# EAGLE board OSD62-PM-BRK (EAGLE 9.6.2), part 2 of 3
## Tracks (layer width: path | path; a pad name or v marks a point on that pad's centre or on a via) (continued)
GPMC0_ADVN_ALE  (via drill 0.1 pad 0.25) (continued)
  Top 0.076: U1.H25 v45.5,14
  Bottom 0.076: v45.5,14 45.75,14.25 46.18,14.25 46.86,14.94 50.14,14.94 52.12,16.92 52.12,21.11 53.49,22.48 56.39,22.48 57.45,23.55 60.73,23.55 61.34,24.16 69.65,24.16 70.87,25.38 75.29,25.38 76.58,26.67 JP4.31
GPMC0_BE0N_CLE  (via drill 0.1 pad 0.25)
  Top 0.076: U1.J26 v46,13.5
  Bottom 0.076: v46,13.5 47.69,13.5 48.23,12.95 50.44,12.95 50.6,12.8 50.6,12.04 48.39,9.83 48.39,7.24 48.92,6.71 55.02,6.71 56.16,5.56 83.13,5.56 83.97,4.72 83.97,3.2 84.51,2.67 93.85,2.67 JP2.38
GPMC0_BE1N  (via drill 0.1 pad 0.25)
  Top 0.076: U1.K25 v45.5,12.5
  Bottom 0.076: v45.5,12.5 45.75,12.25 47.2,12.25 48.08,11.36 48.08,7.09 48.77,6.4 54.86,6.4 56.01,5.26 82.98,5.26 83.67,4.57 83.67,3.05 84.35,2.36 89.08,2.36 JP2.36
GPMC0_CLK  (via drill 0.1 pad 0.25)
  Top 0.076: U1.K26 v46,12.5
  Bottom 0.076: v46,12.5 47.17,12.5 48.23,11.44 48.23,7.16 48.84,6.55 54.94,6.55 56.08,5.41 83.06,5.41 83.82,4.65 83.82,3.12 84.43,2.52 91.47,2.52 JP2.37
GPMC0_CSN0  (via drill 0.1 pad 0.25)
  Top 0.076: U1.F26 v46,15
  Bottom 0.076: v46,15 46.24,15 46.63,15.39 49.91,15.39 51.66,17.14 51.66,21.34 53.26,22.94 56.16,22.94 57.23,24 60.5,24 61.11,24.61 69.42,24.61 71.48,26.67 JP4.29
GPMC0_CSN1  (via drill 0.1 pad 0.25)
  Top 0.076: U1.F25 v45.5,15
  Bottom 0.076: v45.5,15 45.75,15.25 46.26,15.25 46.56,15.54 49.84,15.54 51.51,17.22 51.51,21.41 53.19,23.09 56.08,23.09 57.15,24.16 60.43,24.16 61.04,24.77 69.34,24.77 71.17,26.59 71.17,28.04 72.34,29.21 JP5.29
GPMC0_CSN2  (via drill 0.1 pad 0.25)
  Top 0.076: U1.E26 v46,15.5
  Bottom 0.076: v46,15.5 46.28,15.5 46.48,15.7 49.76,15.7 51.36,17.3 51.36,21.49 53.11,23.24 56.01,23.24 57.07,24.31 60.35,24.31 60.96,24.92 68.12,24.92 69.85,26.64 JP4.28
GPMC0_CSN3  (via drill 0.1 pad 0.25)
  Top 0.076: U1.E25 v45.5,15.5
  Bottom 0.076: v45.5,15.5 45.76,15.76 46.25,15.76 46.34,15.85 49.68,15.85 51.21,17.37 51.21,21.57 53.03,23.39 55.93,23.39 57,24.46 60.27,24.46 60.88,25.07 68.05,25.07 68.66,25.68 68.66,28.04 69.83,29.21 JP5.28
GPMC0_DIR  (via drill 0.1 pad 0.25)
  Top 0.076: U1.G25 v45.5,14.5
  Bottom 0.076: v45.5,14.5 45.75,14.75 46.22,14.75 46.71,15.24 49.99,15.24 51.82,17.07 51.82,21.26 53.34,22.78 56.24,22.78 57.3,23.85 60.58,23.85 61.19,24.46 69.52,24.46 70.74,25.68 72.87,25.68 73.86,26.67 JP4.30
GPMC0_OEN_REN  (via drill 0.1 pad 0.25)
  Top 0.076: U1.H26 v46,14
  Bottom 0.076: v46,14 46.16,14 46.94,14.78 50.22,14.78 52.27,16.84 52.27,21.03 53.57,22.33 56.46,22.33 57.53,23.39 60.81,23.39 61.42,24 69.72,24 70.94,25.22 77.95,25.22 79.4,26.67 JP4.32
GPMC0_WAIT0  (via drill 0.1 pad 0.25)
  Top 0.076: U1.L25 v45.5,12
  Bottom 0.076: v45.5,12 45.75,11.75 47.24,11.75 47.78,11.21 47.78,6.93 48.62,6.1 54.71,6.1 55.85,4.95 80.92,4.95 81.46,4.42 81.46,3.12 81.84,2.74 83.52,2.74 84.99,1.27 JP2.34
GPMC0_WAIT1  (via drill 0.1 pad 0.25)
  Top 0.076: U1.L26 v46,12
  Bottom 0.076: v46,12 47.22,12 47.93,11.29 47.93,7.01 48.69,6.25 54.79,6.25 55.93,5.11 82.91,5.11 83.52,4.5 83.52,2.97 84.28,2.21 86.69,2.21 JP2.35
GPMC0_WEN  (via drill 0.1 pad 0.25)
  Top 0.076: U1.J25 v45.5,13.5
  Bottom 0.076: v45.5,13.5 45.75,13.75 47.67,13.75 48.31,13.11 50.52,13.11 50.75,12.88 50.75,11.96 48.54,9.75 48.54,7.32 49,6.86 55.09,6.86 56.24,5.71 83.21,5.71 84.12,4.8 84.12,3.28 84.58,2.82 96.24,2.82 JP2.39
GPMC0_WPN  (via drill 0.1 pad 0.25)
  Top 0.076: U1.G26 v46,14.5
  Bottom 0.076: v46,14.5 46.2,14.5 46.79,15.09 50.06,15.09 51.97,16.99 51.97,21.18 53.42,22.63 56.31,22.63 57.38,23.7 60.66,23.7 61.27,24.31 69.58,24.31 70.8,25.53 75.21,25.53 76.12,26.44 76.12,28.73 76.61,29.21 JP5.31
I2C0_SCL  (via drill 0.1 pad 0.25, 0.25 pad 0.46)
  Top 0.076: U1.A12 38.75,17.95 39.7,18.9 v40.08,18.9 40.23,18.75 40.84,18.75 42.14,20.04 42.14,20.65 44.27,22.78 51.51,22.78 54.86,19.43 v54.86,19.2 | v74.45,19.96 73.96,20.45 U4.1 | U8.5 77.47,19.75 76.92,19.2 76.05,19.2 75.82,19.43 v75.82,19.96 | v15.47,4.72 14.71,4.72 14.25,5.18 14.25,7.85 14.1,8 v13.64,8
  Top 0.127: U6.10 14.75,12.17 14.35,12.57 v14.35,13.21 14.1,13.46 13.84,13.46 13.72,13.34 13.72,13.03 R52.1 | U7.5 2.46,7.95 2.41,8 2.41,9.4 v2.67,9.65
  Bottom 0.076: v40.08,18.9 39.85,18.9 38.1,20.65 22.55,20.65 20.19,18.29 20.19,16.38 19.74,15.93 15.24,15.93 14.78,15.47 14.78,14.02 14.35,13.59 v14.35,13.21 | v54.86,19.2 54.86,19.81 55.17,20.12 74.3,20.12 v74.45,19.96 74.6,20.12 75.67,20.12 v75.82,19.96 75.97,20.12 97.46,20.12 99.14,21.79 99.14,23.93 99.34,24.13 J7.2 | v14.35,13.21 14.35,12.83 13.34,11.81 13.34,8.31 v13.64,8 | v15.47,4.72 15.67,4.93 20.02,4.93 20.27,5.18 20.27,5.41 19.96,5.72 J8.2 | v14.35,13.21 12.9,13.21 11.12,11.43 8,11.43 7.77,11.66 4.42,11.66 3.96,11.2 3.96,9.6 3.58,9.22 3.1,9.22 v2.67,9.65
I2C0_SDA  (via drill 0.1 pad 0.25, 0.25 pad 0.46)
  Top 0.076: U1.B12 38.5,17 38.5,17.93 39.78,19.2 40.31,19.2 v40.46,19.05 40.62,18.9 40.77,18.9 41.99,20.12 41.99,20.73 44.2,22.94 51.59,22.94 55.17,19.36 55.17,19.13 v54.86,18.82 | U4.3 71.92,20.42 v71.4,20.42 | v75.82,20.42 76.3,20.42 U8.6 | v15.47,4.34 14.86,4.34 14.1,5.11 14.1,7.54 v13.95,7.7
  Top 0.127: U6.9 15.11,12.69 15.11,13.21 v14.77,13.55 v14.35,13.97 R53.1 | U7.6 3.3,8.94 v3.3,9.65
  Bottom 0.076: v40.46,19.05 40.31,19.2 39.78,19.2 38.18,20.8 22.48,20.8 20.04,18.36 20.04,16.46 19.66,16.08 15.16,16.08 14.63,15.54 14.63,14.25 v14.35,13.97 13.44,13.97 11.05,11.58 8.08,11.58 7.85,11.81 4.34,11.81 3.81,11.28 3.81,10.16 v3.3,9.65 | v54.86,18.82 54.56,19.13 54.56,19.96 54.86,20.27 71.25,20.27 v71.4,20.42 71.55,20.27 75.67,20.27 v75.82,20.42 75.97,20.27 97.38,20.27 98.98,21.87 98.98,23.93 98.78,24.13 J7.1 | v14.77,13.55 14.77,13.02 13.49,11.73 13.49,8.53 13.95,8.08 v13.95,7.7 | v15.47,4.34 15.9,4.78 20.1,4.78 20.43,5.1 20.43,6.46 J8.3
I2C1_SCL
  Top 0.076: JP3.36 91.31,4.95 93.34,4.95 93.65,5.26 96.01,5.26 96.55,5.79 96.55,6.93 93.42,10.06 87.94,10.06 87.33,10.67 87.33,18.44 86.49,19.28 81.08,19.28 80.24,18.44 80.24,16.69 79.7,16.15 56.39,16.15 54.41,18.14 54.41,19.43 51.36,22.48 44.42,22.48 42.44,20.5 42.44,19.89 41,18.44 39.7,18.44 39.25,17.99 U1.A13
  Bottom 0.127: JP3.36 R69.1
I2C1_SDA
  Top 0.076: JP3.35 88.77,2.67 90.91,2.67 91.44,3.2 91.44,4.12 92.13,4.8 93.42,4.8 93.73,5.11 96.09,5.11 96.7,5.71 96.7,7.01 93.5,10.21 88.01,10.21 87.48,10.74 87.48,18.52 86.56,19.43 81,19.43 80.09,18.52 80.09,16.76 79.63,16.31 56.46,16.31 54.56,18.21 54.56,19.51 51.44,22.63 44.35,22.63 42.29,20.57 42.29,19.96 40.92,18.59 39.62,18.59 39,17.97 39,17 U1.B13
  Bottom 0.127: JP3.35 R70.1
LDO1-1P8-3P3  (via drill 0.1 pad 0.25, 0.25 pad 0.46)
  Top 0.152: U1.G21 v43.5,14.5 | U1.G22 v44,14.5
  Top 0.254: U6.7 16.28,13.57 v15.62,14.22 15.11,14.73 C42.1 | R43.2 95.17,5.84 94.31,5.84 R44.2 94.16,5.84 93.29,5.84 R45.2 93.22,5.46 92.96,5.21 91.44,5.21 91.19,5.46 R46.2 91.11,5.84 90.25,5.84 R47.2 90.17,5.46 89.66,4.95 87.38,4.95 v86.74,5.59 | v66.06,8.08 65.35,7.37 59.56,7.37 59.05,7.87 53.72,7.87 50.04,11.56 50.04,11.86 C23.1 49.66,11.94 v49.4,12.19
  Route15 0.076: v44,14.5 43.88,14.5 43.75,14.62 43.75,15.12 43.62,15.25 42.38,15.25 42.12,15 | 42.12,15 42.38,14.75 43.25,14.75 v43.5,14.5 U1.G21 42.38,14.25 42.12,14.5 42.12,15
  Route15 0.254: v33.1,17.78 33.1,17.42 33.68,16.84 38.81,16.84 39.37,17.4 39.63,17.4 39.88,17.15 39.88,15.25 40.12,15 42.12,15
  Bottom 0.254: v43.5,14.5 v44,14.5 44.62,13.88 44.62,13.25 44.88,13 47.2,13 48.01,12.19 v49.4,12.19 | v15.62,14.22 16.71,15.32 19.96,15.32 22.85,18.2 32.23,18.2 32.65,17.78 v33.1,17.78 | v86.74,5.59 83.82,5.59 80.77,8.64 66.62,8.64 v66.06,8.08
  pour Route15: 43.38,14.38 43.38,14.62 44.12,14.62 44.12,14.38
LDO2-0P85  (via drill 0.1 pad 0.25, 0.25 pad 0.46)
  Top 0.076: C18.1 15.39,8.76 15.57,8.94 16.67,8.94 16.78,8.83 U6.19
  Top 0.152: U1.K17 v41.5,12.5 | U1.L17 v41.5,12 | U1.L18 v42,12 | U1.K18 v42,12.5 | U1.H17 v41.5,14 | U1.J17 v41.5,13.5 | U1.J18 v42,13.5 | U1.H18 v42,14 | v20.73,5.77 20.88,5.92 21,5.92 C17.1 | C19.1 40.16,7.39 v40.01,7.54
  Top 0.254: C43.1 15.75,7.49 15.88,7.62 v16.26,7.62 16.78,8.14 U6.19
  Route15 0.152: v20.73,5.77 20.73,6.38
  Route15 0.381: v16.26,7.62 17.5,6.38 19.94,6.38 20.73,6.38 34.19,6.38 37.34,9.53 38.86,9.53 41.34,12 v41.5,12
  Bottom 0.152: v41.5,12 41.16,11.66 40.39,11.66 40.16,11.89 39.85,11.89 39.62,11.66 39.62,11.35 39.78,11.2 39.78,10.75 39.17,10.13 39.17,7.71 39.49,7.39 39.85,7.39 v40.01,7.54
  pour Route15: 41.38,14.12 41.38,12.25 40.62,11.5 41.62,11.5 42.12,12 42.12,14.12
LDO3-1P8  (via drill 0.1 pad 0.25, 0.25 pad 0.46)
  Top 0.076: U1.D15 v40.5,16
  Top 0.127: R24.2 14.73,6.35 14.86,6.48 17.65,6.48 | 17.78,6.6 17.65,6.48 | 17.78,6.6 C44.1 | Y1.4 29.11,17.88 28.7,18.29 28.7,18.31 C46.1 | 17.78,6.6 17.91,6.48 | C5.1 21.29,6.48 17.91,6.48 | 17.65,6.48 17.91,6.48
  Top 0.152: U1.P11 v38,10.5 | U1.N12 v38.5,11 | U1.N13 v39,11 | U1.P12 v38.5,10.5 | U1.P13 v39,10.5 | U1.N14 v39.5,11 | U1.F13 v39,15 | U1.F14 v39.5,15 | v24.08,19.81 24.69,19.2 24.69,16.92 v24.92,16.69 | 28.7,18.31 28.63,18.39 28.6,18.36 27.61,18.36 27.2,18.77 v27.2,19.81 27.2,20.8 | 27.2,20.8 27.64,20.8 R50.1 27.74,20.8 28.83,20.8 Y2.4 | 27.2,20.8 26.72,20.8 C54.1 | C3.1 39.78,18.14 v39.62,17.98 | C4.1 29.72,7.49 | 29.72,7.49 v29.72,7.47 | C1.1 30.48,7.92 30.05,7.49 29.72,7.49 | C2.1 41.07,7.39 v41.22,7.54
  Top 0.254: C44.1 v17.78,7.67 U6.21
  Route15 0.381: v38.5,10.5 38.03,10.03 37.16,10.03 34.01,6.88 30.91,6.88 30.33,7.47 v29.72,7.47 29.11,7.47 28.52,6.88 18.26,6.88 17.78,7.37 v17.78,7.67
  Bottom 0.152: v39,15 v39.5,15 39.75,15 40.5,15.75 v40.5,16 40,16.5 40,17.45 39.62,17.83 | v24.08,19.81 v27.2,19.81 37.64,19.81 39.47,17.98 | v24.92,16.69 23.39,16.69 22.4,15.7 22.4,13.41 21.26,12.27 19.58,12.27 18.75,11.43 16.38,11.43 16,11.05 16,8.43 16.64,7.8 16.64,7.52 16.99,7.16 17.27,7.16 v17.78,7.67 | v39,10.5 38.92,10.42 38.92,7.63 39.4,7.16 40.84,7.16 v41.22,7.54 | 39.47,17.98 v39.62,17.98 39.62,17.83 | 39.47,17.98 39.62,17.83
  pour Route15: 38.5,11.12 37.28,9.91 38.66,9.91 39.88,11.12
LDO4-2P5  (via drill 0.1 pad 0.25, 0.25 pad 0.46)
  Top 0.152: U1.N10 v37.5,11 | C20.1 v30.35,11.56
  Top 0.254: U6.23 18.78,8.28 v19.43,7.62 19.68,7.62 19.81,7.49 C45.1
  Route15 0.254: v37.5,11 37.5,10.98 33.83,7.32 31.09,7.32 30.48,7.92 28.96,7.92 28.35,7.32 19.74,7.32 v19.43,7.62
  Bottom 0.076: v37.5,11 37.25,11.25 33.8,11.25 33.3,10.74 32.54,10.74 31.73,11.56 v30.35,11.56
LED1
  Top 0.127: R57.1 3.25,21.08 2.27,21.08 D1.1
LED2
  Top 0.076: R58.1 82.68,16.76 82.45,16.54 82.22,16.54 81.61,15.93 81.61,11.94 81.86,11.68 D2.1
LED3
  Top 0.076: R59.1 81.66,16.2 81.46,16 81.46,10.11 81.79,9.78 D3.1
LED4
  Top 0.076: R60.1 83.69,16.64 83.44,16.38 82.3,16.38 81.76,15.85 81.76,13.72 81.89,13.59 D4.1
LED5
  Top 0.076: D5.1 82.44,16.07 82.6,16.23 84.35,16.23 84.71,16.59 R61.1
LX_B1
  pour Top (no thermals): 18.16,13.08 18.16,13.97 19.05,14.86 19.05,16.13 20.07,16.13 20.07,14.22 19.43,14.22 18.92,13.72 18.92,13.08
LX_B2
  pour Top (no thermals): 19.68,11 21.84,11 21.84,12.06 21.03,12.06 21.03,11.33 19.68,11.33
LX_B3
  pour Top (no thermals): 19.68,10.34 21.84,10.34 21.84,9.27 21.01,9.27 21.01,10.06 19.68,10.06
MCAN0_RX
  Top 0.076: U1.A11 38.25,17.91 39.7,19.36 40.98,19.36 41.83,20.21 41.83,20.8 44.12,23.09 51.66,23.09 58.29,16.46 79.55,16.46 79.93,16.84 79.93,18.59 80.92,19.58 86.64,19.58 87.63,18.59 87.63,10.82 88.09,10.36 93.57,10.36 96.85,7.09 96.85,5.64 96.16,4.95 93.8,4.95 92.71,3.86 JP3.37
MCAN0_TX
  Top 0.076: U1.B11 38,17 38,17.88 39.62,19.51 40.92,19.51 41.68,20.27 41.68,20.88 44.04,23.24 51.74,23.24 58.37,16.61 79.48,16.61 79.78,16.92 79.78,18.67 80.85,19.74 86.72,19.74 87.78,18.67 87.78,10.9 88.16,10.52 93.65,10.52 97,7.16 97,5.56 JP3.38
MCASP0_ACLKR  (via drill 0.1 pad 0.25)
  Top 0.076: U1.B19 42.5,17 42.5,17.66 43.81,18.97 43.81,19.81 44.81,20.8 50.37,20.8 55.93,15.24 80.09,15.24 81.15,14.17 81.15,9.6 81.69,9.07 93.95,9.07 95.78,7.24 v95.78,5.79
  Bottom 0.076: v95.78,5.79 97.77,3.81 JP3.39
MCASP0_ACLKX
  Top 0.076: U1.A18 41.75,17.59 43.36,19.2 43.36,20.04 44.58,21.26 50.6,21.26 56.16,15.7 79.93,15.7 80.7,16.46 80.7,18.21 81.31,18.82 82.58,18.82 82.68,18.72 R58.2
MCASP0_AFSR  (via drill 0.1 pad 0.25)
  Top 0.076: v96.09,6.1 95.94,6.25 95.94,7.32 95.86,7.39 94.03,9.22 81.76,9.22 81.31,9.68 81.31,14.25 80.16,15.39 56.01,15.39 50.44,20.95 44.73,20.95 43.66,19.89 43.66,19.05 42.25,17.64 U1.A19
  Bottom 0.076: v96.09,6.1 96.09,5.71 96.85,4.95 99.19,4.95 JP3.40
MCASP0_AFSX
  Top 0.076: U1.B18 42,17 42,17.62 43.51,19.13 43.51,19.96 44.65,21.11 50.52,21.11 56.08,15.54 80.01,15.54 80.85,16.38 80.85,17.98 81.2,18.34 R59.2
MCASP0_AXR0
  Top 0.076: U1.B17 41.5,17 41.5,17.57 43.2,19.28 43.2,20.12 44.5,21.41 50.67,21.41 56.24,15.85 79.86,15.85 80.54,16.54 80.54,18.29 81.23,18.97 83.52,18.97 83.69,18.8 R60.2
MCASP0_AXR1
  Top 0.076: U1.A17 41.25,17.55 43.05,19.36 43.05,20.19 44.42,21.57 50.75,21.57 56.31,16 79.78,16 80.39,16.61 80.39,18.36 81.15,19.13 84.43,19.13 84.71,18.85 R61.2
MCASP0_AXR2  (via drill 0.1 pad 0.25)
  Top 0.076: U1.B16 41,17 41,17.53 42.9,19.43 42.9,20.27 44.35,21.72 50.83,21.72 53.65,18.9 v53.8,18.9
  Bottom 0.076: v53.8,18.9 53.65,19.05 53.65,19.89 54.48,20.73 69.42,20.73 71.63,22.94 84.35,22.94 86.64,25.22 94.03,25.22 94.41,25.6 96.77,25.6 97.79,26.62 JP4.39
MCASP0_AXR3  (via drill 0.1 pad 0.25)
  Top 0.076: v54.1,18.67 54.1,18.97 51.21,21.87 44.27,21.87 42.75,20.34 42.75,19.51 40.75,17.51 U1.A16 | v95.91,25.3 95.91,24.71 R55.1
  Bottom 0.076: v54.1,18.67 54.1,18.97 53.8,19.28 53.8,19.81 54.56,20.57 69.49,20.57 71.7,22.78 84.43,22.78 86.72,25.07 94.11,25.07 94.49,25.45 95.76,25.45 v95.91,25.3
MCU_ERRORN  (via drill 0.1 pad 0.25)
  Top 0.076: U1.D7 v36,16
  Bottom 0.076: TP2.TP U1.D7 v36,16
MCU_I2C0_SCL  (via drill 0.1 pad 0.25)
  Top 0.076: U1.A7 36.25,17.39 35.74,17.91 35.74,22.86 35.94,23.06 35.94,23.37 36.14,23.57 R65.1 36.45,24 36.32,24.13 v35.94,24.13
  Bottom 0.076: v35.94,24.13 35.74,24.33 35.74,27.76 JP5.14
MCU_I2C0_SDA  (via drill 0.1 pad 0.25)
  Top 0.076: U1.B7 36,17 36,17.42 35.59,17.83 35.59,22.94 35.43,23.09 R66.1 v35.43,24.13
  Bottom 0.076: v35.43,24.13 35.13,24.43 35.13,25.83 JP4.14
MCU_MCAN0_RX
  Top 0.076: U1.E1 32.75,15.25 31.93,16.07 31.93,21.34 31.55,21.72 25.15,21.72 22.1,24.77 19.28,24.77 17.91,26.14 17.91,27.28 17.22,27.96 15.85,27.96 15.7,28.12 13.34,28.12 13.18,28.27 10.9,28.27 9.96,29.21 JP5.4
MCU_MCAN0_TX
  Top 0.076: U1.E2 33.5,15.5 32.75,15.5 32.08,16.17 32.08,21.41 31.62,21.87 25.22,21.87 22.17,24.92 19.36,24.92 18.06,26.21 18.06,27.36 17.3,28.12 15.93,28.12 15.77,28.27 13.41,28.27 12.47,29.21 JP5.5
MCU_MCAN1_RX
  Top 0.076: U1.F1 32.75,14.75 31.62,15.88 31.62,21.18 31.39,21.41 24.99,21.41 21.95,24.46 19.13,24.46 17.6,25.98 17.6,27.13 17.07,27.66 15.7,27.66 15.54,27.81 13.18,27.81 13.03,27.96 5.11,27.96 3.86,29.21 JP5.2
MCU_MCAN1_TX
  Top 0.076: U1.F2 33.5,15 32.75,15 31.77,15.97 31.77,21.26 31.47,21.57 25.07,21.57 22.02,24.61 19.2,24.61 17.75,26.06 17.75,27.2 17.14,27.81 15.77,27.81 15.62,27.96 13.26,27.96 13.11,28.12 7.47,28.12 6.38,29.21 JP5.3
MCU_OSC0_XI
  Top 0.076: U1.G1 32.84,14.25 31.39,15.7 31.39,20.34 30.94,20.8 30.35,20.8 Y2.3
MCU_PORZ  (via drill 0.1 pad 0.25)
  Top 0.076: U1.D6 v35.5,16 | v35.33,18.29 35.43,18.39 35.43,22.39 v35.34,22.48
  Top 0.127: U6.18 16.28,8.15 16.13,8 14.99,8 v14.73,7.75 R24.1
  Bottom 0.076: v35.5,16 35.25,16.25 35.25,17.98 35.33,18.06 v35.33,18.29 35.18,18.44 22.71,18.44 19.89,15.62 15.47,15.62 15.24,15.39 15.24,12.88 14.73,12.37 v14.73,7.75 | 36.42,26.26 JP4.15 36.04,25.88 36.04,25.22 36.42,24.84 36.42,22.78 36.12,22.48 v35.34,22.48
MCU_RESETSTATZ  (via drill 0.1 pad 0.25)
  Top 0.076: U1.C6 v35.5,16.5
  Bottom 0.076: TP3.TP 35.62,15 35.75,15.12 U1.C6 v35.5,16.5
MCU_RESETZ  (via drill 0.1 pad 0.25)
  Top 0.076: U1.C5 v35,16.5 | v33.68,17.83 33.53,17.83 33.4,17.96 R10.1
  Bottom 0.076: v35,16.5 35,17.27 34.44,17.83 v33.68,17.83
MCU_SPI0_CLK
  Top 0.076: U1.A4 34.75,17.52 34.44,17.83 34.44,24.77 34.14,25.07 32.46,25.07 32.31,25.22 28.12,25.22 JP4.11
MCU_SPI0_CS0
  Top 0.076: U1.B6 35.5,17 35.5,17.46 34.9,18.06 34.9,24.99 34.37,25.53 32.69,25.53 32.54,25.68 31.24,25.68 30.63,26.29 30.63,28.09 JP5.13
MCU_SPI0_CS1
  Top 0.076: U1.A6 35.75,17.44 35.05,18.14 35.05,25.07 34.44,25.68 32.77,25.68 31.77,26.67 JP4.13
MCU_SPI0_D0
  Top 0.076: U1.B5 35,17 35,17.5 34.59,17.91 34.59,24.84 34.21,25.22 32.54,25.22 32.38,25.38 28.88,25.38 28.12,26.14 28.12,28.12 JP5.12
MCU_SPI0_D1
  Top 0.076: U1.A5 35.25,17.48 34.75,17.98 34.75,24.92 34.29,25.38 32.61,25.38 32.46,25.53 30.33,25.53 29.21,26.64 JP4.12
MCU_UART0_CTSN
  Top 0.076: U1.B4 34.5,17 34.5,17.55 34.29,17.75 34.29,21.26 32.46,23.09 25.83,23.09 25.38,23.55 25.38,27.91 JP5.11
MCU_UART0_RTSN
  Top 0.076: U1.A3 34.25,17.57 34.14,17.68 34.14,21.18 32.38,22.94 25.76,22.94 24.13,24.56 JP4.10
MCU_UART0_RXD
  Top 0.076: U1.B2 32.84,17.66 32.84,21.79 32,22.63 25.6,22.63 21.59,26.64 JP4.9
MCU_UART0_TXD
  Top 0.076: U1.B3 34,17 34,17.59 33.98,17.6 33.98,21.11 32.31,22.78 25.68,22.78 23.01,25.45 23.01,28.09 JP5.10
MDIO0_MDC
  Top 0.076: JP3.12 30.35,2.67 44.88,2.67 45.75,3.54 U1.V26
MDIO0_MDIO
  Top 0.076: U1.U26 46,9 46,3.56 44.96,2.52 30.45,2.52 JP2.12
MMC0_CLK
  Top 0.076: JP4.5 12.42,27.66 14.86,27.66 15.24,27.28 15.24,26.06 15.77,25.53 17.83,25.53 19.05,24.31 21.87,24.31 26.14,20.04 26.14,18.44 29.87,14.71 31.47,14.71 32.93,13.25 U1.J1
  Bottom 0.127: R67.1 JP4.5
MMC0_CMD
  Top 0.076: U1.K1 33.02,12.75 32.97,12.8 31.55,12.8 25.98,18.36 25.98,19.96 21.79,24.16 18.97,24.16 17.75,25.38 15.24,25.38 13.97,26.64 JP4.6
  Bottom 0.127: R68.1 JP4.6
MMC0_DAT0  (via drill 0.1 pad 0.25)
  Top 0.076: U1.K2 33.5,12.5 32.99,12.5 32.84,12.65 32.69,12.65 v32.38,12.34
  Bottom 0.076: JP3.4 9.98,3.81 11.12,4.95 14.63,4.95 15.47,5.79 15.47,12.19 16.08,12.8 20.34,12.8 21.87,14.33 21.87,15.93 23.24,17.3 27.43,17.3 27.89,16.84 31.93,16.84 32.23,16.54 32.23,12.5 v32.38,12.34
MMC0_DAT1  (via drill 0.1 pad 0.25)
  Top 0.076: v32.77,12.34 32.99,12.34 33.09,12.25 U1.L1
  Bottom 0.076: JP3.3 7.34,4.8 10.74,4.8 11.05,5.11 14.55,5.11 15.32,5.87 15.32,12.27 16,12.95 20.27,12.95 21.72,14.4 21.72,16 23.16,17.45 27.51,17.45 27.96,16.99 32,16.99 32.38,16.61 32.38,12.72 v32.77,12.34
MMC0_DAT2
  Top 0.076: U1.L2 33.5,12 33.03,12 32.99,12.04 32.08,12.04 25.83,18.29 25.83,19.89 21.72,24 18.9,24 17.68,25.22 10.82,25.22 10.13,25.91 10.13,27.36 9.68,27.81 3.5,27.81 2.36,26.67 JP4.1
MMC0_DAT3
  Top 0.076: U1.M1 33.06,11.75 32.92,11.89 32,11.89 25.68,18.21 25.68,19.81 21.64,23.85 18.82,23.85 17.6,25.07 10.74,25.07 9.98,25.83 9.98,27.28 9.6,27.66 4.88,27.66 3.89,26.67 JP4.2
MMC0_DAT4  (via drill 0.1 pad 0.25)
  Top 0.076: U1.M2 33.5,11.5 33.08,11.5 32.84,11.73 32.61,11.73 v32.46,11.58
  Bottom 0.076: JP3.6 15.77,5.61 15.77,12.04 16.23,12.5 20.5,12.5 22.17,14.17 22.17,15.77 23.39,16.99 27.28,16.99 27.74,16.54 31.77,16.54 31.93,16.38 31.93,12.12 v32.46,11.58
MMC0_DAT5  (via drill 0.1 pad 0.25)
  Top 0.076: v32.77,11.35 32.87,11.25 U1.N1
  Bottom 0.076: JP3.5 12.42,4.8 14.71,4.8 15.62,5.71 15.62,12.12 16.15,12.65 20.42,12.65 22.02,14.25 22.02,15.85 23.32,17.14 27.36,17.14 27.81,16.69 31.85,16.69 32.08,16.46 32.08,12.19 32.38,11.89 32.54,11.89 32.77,11.66 v32.77,11.35
MMC0_DAT6
  Top 0.076: U1.N2 33.5,11 32.66,11 25.53,18.14 25.53,19.74 21.57,23.7 18.75,23.7 17.53,24.92 10.67,24.92 8.91,26.67 JP4.4
MMC0_DAT7
  Top 0.076: U1.P1 32.68,10.75 25.38,18.06 25.38,19.66 21.49,23.55 18.67,23.55 17.45,24.77 9.22,24.77 7.32,26.67 JP4.3
MMC1_CLK
  Top 0.076: U1.B21 43.5,17 43.5,17.59 44.42,18.52 44.42,19.51 45.11,20.19 50.06,20.19 55.63,14.63 79.78,14.63 80.54,13.87 80.54,9.3 81.38,8.46 90.75,8.46 91.67,7.54 91.67,6.1 91.85,5.92 R33.2
MMC1_CLK_R  (via drill 0.1 pad 0.25, 0.25 pad 0.46)
  Top 0.076: R33.1 v92.2,6.48
  Top 0.127: 96.42,12.7 95.38,12.7 95.25,12.83 95.25,13.21 95.12,13.34 94.74,13.34 94.61,13.21 94.61,12.83 94.49,12.7 94.11,12.7 93.98,12.83 93.98,13.21 93.85,13.34 93.47,13.34 93.34,13.21 93.34,12.83 93.22,12.7 92.84,12.7 92.71,12.83 92.71,13.21 92.58,13.34 92.2,13.34 92.08,13.21 92.08,12.83 91.95,12.7 v91.69,12.7
  Top 0.152: X1.PIN5 96.42,12.7
  Bottom 0.127: v91.69,12.7 91.69,6.99 v92.2,6.48
MMC1_CMD  (via drill 0.1 pad 0.25, 0.25 pad 0.46)
  Top 0.076: U1.A21 43.25,17.57 44.27,18.59 44.27,19.58 45.03,20.34 50.14,20.34 55.7,14.78 79.86,14.78 80.7,13.95 80.7,9.37 81.46,8.61 92.2,8.61 93.22,7.59 R45.1 v93.22,6.48
  Top 0.127: X1.PIN3 95.38,14.99 95.25,15.11 95.25,15.49 95.12,15.62 94.74,15.62 94.61,15.49 94.61,15.11 94.49,14.99 94.11,14.99 93.98,15.11 93.98,15.49 93.85,15.62 93.47,15.62 93.34,15.49 93.34,15.11 93.22,14.99 v92.2,14.99
  Bottom 0.127: v92.2,14.99 92.71,14.48 92.71,6.99 v93.22,6.48
MMC1_DAT0  (via drill 0.1 pad 0.25, 0.25 pad 0.46)
  Top 0.076: U1.A22 43.75,17.61 44.58,18.44 44.58,19.43 45.19,20.04 49.99,20.04 55.55,14.48 79.7,14.48 80.39,13.79 80.39,9.22 81.31,8.31 90.45,8.31 91.19,7.57 R46.1 v91.19,6.48
  Top 0.127: X1.PIN7 96.46,10.54 95.5,10.54 95.25,10.79 95.25,12.32 95.12,12.45 94.74,12.45 94.61,12.32 94.61,11.94 94.49,11.81 94.11,11.81 93.98,11.94 93.98,12.32 93.85,12.45 93.47,12.45 93.34,12.32 93.34,11.94 93.22,11.81 92.84,11.81 92.71,11.94 92.71,12.32 92.58,12.45 92.2,12.45 92.08,12.32 92.08,11.94 91.95,11.81 91.57,11.81 90.68,12.7 v90.68,13.08
  Bottom 0.127: v90.68,13.08 90.68,6.73 90.93,6.48 v91.19,6.48
MMC1_DAT1  (via drill 0.1 pad 0.25, 0.25 pad 0.46)
  Top 0.076: U1.B22 44,17 44,17.64 44.73,18.36 44.73,19.36 45.26,19.89 49.91,19.89 55.47,14.33 79.63,14.33 80.24,13.72 80.24,9.14 81.23,8.15 89.61,8.15 90.17,7.59 R47.1 90.17,6.6 90.04,6.48 v89.66,6.48
  Top 0.127: X1.PIN8 96.45,9.53 95.5,9.53 94.61,10.41 94.61,11.43 94.49,11.56 94.11,11.56 93.98,11.43 93.98,10.92 93.85,10.79 93.47,10.79 93.34,10.92 93.34,11.43 93.22,11.56 92.84,11.56 92.71,11.43 92.71,10.92 92.58,10.79 92.2,10.79 92.08,10.92 92.08,11.43 91.95,11.56 91.57,11.56 91.44,11.43 91.44,10.92 91.31,10.79 90.93,10.79 90.81,10.92 90.81,11.94 90.68,12.06 90.3,12.06 90.17,11.94 90.17,11.05 90.04,10.92 v89.66,10.92
  Bottom 0.127: v89.66,10.92 v89.66,6.48
MMC1_DAT2  (via drill 0.1 pad 0.25, 0.25 pad 0.46)
  Top 0.076: v95.25,6.48 R43.1 95.25,7.54 93.88,8.91 81.61,8.91 81,9.53 81,14.1 80.01,15.09 55.85,15.09 50.29,20.65 44.88,20.65 43.97,19.74 43.97,18.75 42.75,17.53 U1.A20
  Top 0.127: v94.74,17.27 96.4,17.27 X1.PIN1
  Bottom 0.127: v95.25,6.48 94.74,6.99 v94.74,17.27
MMC1_DAT3  (via drill 0.1 pad 0.25, 0.25 pad 0.46)
  Top 0.076: U1.B20 43,17 43,17.55 44.12,18.67 44.12,19.66 44.96,20.5 50.22,20.5 55.78,14.94 79.93,14.94 80.85,14.02 80.85,9.45 81.53,8.76 93.04,8.76 94.23,7.57 R44.1 v94.23,6.48
  Top 0.127: X1.PIN2 96.25,16.13 95.38,16.13 95.25,16.26 95.25,16.51 95.12,16.64 94.74,16.64 94.61,16.51 94.61,16.26 94.49,16.13 v93.73,16.13
  Bottom 0.127: v93.73,16.13 93.73,6.99 v94.23,6.48
MMC1_SDCD
  Top 0.076: U1.A23 44.25,17.66 44.88,18.29 44.88,19.28 45.34,19.74 49.84,19.74 55.4,14.17 79.4,14.17 80.09,13.49 80.09,9.07 81.15,8 88.85,8 89.25,7.6 U11.4
MMC1_SDWP  (via drill 0.1 pad 0.25)
  Top 0.076: U1.B23 44.5,17 44.5,17.37 v46.1,18.97 | R13.1 13.23,10.92 13.11,11.05 13.11,14.25 13.41,14.55 v14.33,14.55
  Top 0.127: U6.12 14.48,11.18 14.22,11.43 13.84,11.43 13.72,11.3 13.72,11 R13.1
  Bottom 0.076: v14.33,14.55 14.48,14.71 14.48,15.62 15.09,16.23 19.2,16.23 19.43,16.46 19.43,18.21 22.33,21.11 37.57,21.11 38.02,21.57 38.02,24.99 38.48,25.45 42.9,25.45 43.59,24.77 46.48,24.77 46.86,24.38 46.86,20.04 46.1,19.28 v46.1,18.97
MMC2_CLK  (via drill 0.1 pad 0.25)
  Top 0.076: U1.D23 v44.5,16
  Bottom 0.076: v44.5,16 44.75,16.25 44.75,16.79 45.19,17.22 47.62,17.22 48.39,17.98 48.39,25.53 JP4.20
MMC2_CMD  (via drill 0.1 pad 0.25)
  Top 0.076: U1.C23 v44.5,16.5
  Bottom 0.076: v44.5,16.5 44.5,16.84 45.41,17.75 47.32,17.75 48.23,18.67 48.23,28.04 49.4,29.21 JP5.20
MMC2_DAT0  (via drill 0.1 pad 0.25)
  Top 0.076: U1.D22 v44,16
  Bottom 0.076: v44,16 44.25,16.25 44.25,16.82 45.34,17.91 47.24,17.91 48.08,18.75 48.08,28.04 46.99,29.13 JP5.19
MMC2_DAT1  (via drill 0.1 pad 0.25)
  Top 0.076: U1.C22 v44,16.5
  Bottom 0.076: v44,16.5 44,16.8 45.26,18.06 47.17,18.06 47.93,18.82 47.93,25.73 JP4.19
MMC2_DAT2  (via drill 0.1 pad 0.25)
  Top 0.076: U1.D21 v43.5,16
  Bottom 0.076: v43.5,16 43.75,16.25 43.75,16.77 45.19,18.21 47.09,18.21 47.78,18.9 47.78,24.84 46.94,25.68 46.25,25.68 45.64,26.29 45.64,28.04 44.48,29.21 JP5.18
MMC2_DAT3  (via drill 0.1 pad 0.25)
  Top 0.076: U1.C21 v43.5,16.5
  Bottom 0.076: v43.5,16.5 43.5,16.75 45.11,18.36 47.02,18.36 47.62,18.97 47.62,24.77 46.86,25.53 45.59,25.53 JP4.18
MMC2_SDCD  (via drill 0.1 pad 0.25)
  Top 0.076: U1.D20 v43,16
  Bottom 0.076: v43,16 43.25,16.25 43.25,16.73 45.03,18.52 46.94,18.52 47.47,19.05 47.47,24.69 46.79,25.38 44.35,25.38 43.13,26.59 43.13,28.04 41.96,29.21 JP5.17
MMC2_SDWP  (via drill 0.1 pad 0.25)
  Top 0.076: U1.C20 v43,16.5
  Bottom 0.076: v43,16.5 43,16.71 44.96,18.67 46.86,18.67 47.32,19.13 47.32,24.61 46.71,25.22 44.27,25.22 42.82,26.67 JP4.17
MPU_HFOSC_EN
  Top 0.127: R50.2 27.76,19.56 28.81,19.56 Y2.1
OSPI0_CLK  (via drill 0.1 pad 0.25)
  Top 0.076: U1.A24 44.75,17.39 46.02,18.67 49.45,18.67 v49.61,18.52
  Bottom 0.076: v49.61,18.52 49.84,18.75 49.84,22.25 52.35,24.77 55.24,24.77 JP4.23
OSPI0_CSN0  (via drill 0.1 pad 0.25)
  Top 0.076: U1.D25 v45.5,16
  Bottom 0.076: v45.5,16 45.75,16.25 46.2,16.25 46.41,16.46 48.01,16.46 49.15,17.6 49.15,22.02 52.2,25.07 54.18,25.07 54.61,25.5 JP4.22
OSPI0_CSN1  (via drill 0.1 pad 0.25)
  Top 0.076: U1.C25 v45.5,16.5 | v80.47,24.92 80.31,24.77 D7.CATHODE
  Bottom 0.076: v45.5,16.5 45.76,16.76 47.85,16.76 48.84,17.75 48.84,22.17 52.05,25.38 52.88,25.38 53.34,25.83 53.34,29.57 53.95,30.18 80.92,30.18 81.38,29.72 81.38,25.98 80.47,25.07 v80.47,24.92
OSPI0_CSN2  (via drill 0.1 pad 0.25)
  Top 0.076: U1.D24 v45,16
  Bottom 0.076: v45,16 45.25,16.25 45.25,16.6 45.57,16.92 47.78,16.92 48.69,17.83 48.69,22.25 52.07,25.63 JP4.21
OSPI0_CSN3  (via drill 0.1 pad 0.25)
  Top 0.076: U1.C24 v45,16.5
  Bottom 0.076: v45,16.5 45,16.73 45.34,17.07 47.7,17.07 48.54,17.91 48.54,22.33 50.9,24.69 50.9,28.04 JP5.21
OSPI0_D0  (via drill 0.1 pad 0.25)
  Top 0.076: U1.B24 45,17 45,17.42 46.1,18.52 49,18.52 49.3,18.21 v49.84,18.21
  Bottom 0.076: v49.84,18.21 49.99,18.36 49.99,22.17 52.43,24.61 55.32,24.61 56.39,25.68 57.99,25.68 58.52,26.21 58.52,28.04 JP5.24
OSPI0_D1  (via drill 0.1 pad 0.25)
  Top 0.076: U1.A25 45.25,17.44 46.18,18.36 48.84,18.36 49.3,17.91 v49.99,17.91
  Bottom 0.076: v49.99,17.91 50.14,18.06 50.14,22.1 52.5,24.46 55.4,24.46 56.46,25.53 58.55,25.53 JP4.24
OSPI0_D2  (via drill 0.1 pad 0.25)
  Top 0.076: U1.B25 45.5,17 45.5,17.46 46.25,18.21 48.69,18.21 49.3,17.6 v49.76,17.6
  Bottom 0.076: v49.76,17.6 50.06,17.6 50.29,17.83 50.29,22.02 52.58,24.31 55.47,24.31 56.54,25.38 59.82,25.38 61.04,26.59 61.04,28.04 62.2,29.21 JP5.25
OSPI0_D3  (via drill 0.1 pad 0.25)
  Top 0.076: U1.A26 45.75,17.48 46.33,18.06 48.46,18.06 49.23,17.3 v49.53,17.3
  Bottom 0.076: v49.53,17.3 49.99,17.3 50.44,17.75 50.44,21.95 52.65,24.16 55.55,24.16 56.62,25.22 59.89,25.22 60.5,25.83 61.39,25.83 JP4.25
OSPI0_D4  (via drill 0.1 pad 0.25)
  Top 0.076: U1.B26 46,17 46,17.5 46.41,17.91 48.31,17.91 v49.23,16.99
  Bottom 0.076: v49.23,16.99 49.91,16.99 50.6,17.68 50.6,21.87 52.73,24 55.63,24 56.69,25.07 59.98,25.07 60.59,25.68 63.17,25.68 63.63,26.14 63.63,28.04 64.77,29.18 JP5.26
OSPI0_D5  (via drill 0.1 pad 0.25)
  Top 0.076: U1.B27 47.26,17.75 47.85,17.75 v48.92,16.69
  Bottom 0.076: v48.92,16.69 49.84,16.69 50.75,17.6 50.75,21.79 52.81,23.85 55.7,23.85 56.77,24.92 60.05,24.92 60.66,25.53 63.63,25.53 JP4.26
OSPI0_D6  (via drill 0.1 pad 0.25)
  Top 0.076: U1.C27 46.5,16.5 48.5,16.5 v48.62,16.38
  Bottom 0.076: v48.62,16.38 49.76,16.38 50.9,17.53 50.9,21.72 52.88,23.7 55.78,23.7 56.84,24.77 60.12,24.77 60.73,25.38 65.53,25.38 66.14,25.98 66.14,28.04 JP5.27
OSPI0_D7  (via drill 0.1 pad 0.25)
  Top 0.076: v48.31,16.15 48.16,16.31 47.09,16.31 47.03,16.25 U1.C28
  Bottom 0.076: v48.31,16.15 48.46,16 49.61,16 51.05,17.45 51.05,21.64 52.96,23.55 55.85,23.55 56.92,24.61 60.2,24.61 60.81,25.22 65.84,25.22 67.28,26.67 JP4.27
OSPI0_DQS  (via drill 0.1 pad 0.25)
  Top 0.076: U1.D26 v46,16
  Bottom 0.076: v46,16 46.17,16 46.48,16.31 48.08,16.31 49.3,17.53 49.3,21.95 52.27,24.92 54.79,24.92 56.01,26.14 56.01,28.04 57.15,29.18 JP5.23
OSPI0_LBCLKO  (via drill 0.1 pad 0.25)
  Top 0.076: U1.C26 v46,16.5 | R74.2 53.14,24.64 53.49,24.99 v53.49,25.38
  Bottom 0.076: v46,16.5 46.11,16.61 47.93,16.61 49,17.68 49,22.1 52.12,25.22 53.34,25.22 v53.49,25.38 53.49,28.04 54.61,29.16 JP5.22
OSPI0_LBCLKO_R  (via drill 0.1 pad 0.25)
  Top 0.076: R74.1 50.85,24.64 50.22,24 43.59,24 43.2,24.38 43.2,25.07 42.9,25.38 39.47,25.38 38.99,24.89 J1.1 37.85,24 v37.72,24.13 | v21.95,21.26 22.1,21.11 22.1,19.13 24.84,16.38 25.6,16.38 v25.76,16.54 | U13.C1 27.05,13.84 27.05,14.78 26.98,14.86 26.75,14.86 26.52,15.09 v26.52,15.24
  Bottom 0.076: v37.72,24.13 37.87,23.98 37.87,21.64 37.49,21.26 v21.95,21.26 | v25.76,16.54 26.52,15.77 v26.52,15.24
PMIC_LPM_EN0  (via drill 0.1 pad 0.25)
  Top 0.076: U1.D5 v35,16 | U6.31 19.6,12.17 19.51,12.27 19.51,12.88 19.96,13.34 v19.96,13.56
  Top 0.127: U6.31 20.55,12.17 21.03,12.65 R23.1
  Bottom 0.076: v35,16 34.75,16.25 34.75,16.84 34.52,17.07 33.45,17.07 33.07,17.45 32.54,17.45 32.08,17.91 22.94,17.91 21.26,16.23 21.26,14.63 20.19,13.56 v19.96,13.56
PMIC_PWR_BTN
  Top 0.127: S1.P$1 S1.P$2 28.13,7.04 27.81,6.73 23.88,6.73 23.5,7.11 22.1,7.11 21.97,7.24 21.97,7.49 21.84,7.62 R22.1 19.93,9.11 U6.25
PORZ_OUT  (via drill 0.1 pad 0.25)
  Top 0.076: U1.D18 v42,16
  Bottom 0.076: v42,16 U1.D18 TP1.TP
RESET_REQZ  (via drill 0.1 pad 0.25)
  Top 0.076: U1.D17 v41.5,16 | R11.1 42.67,23.01 42.14,22.48 v41.99,22.48
  Bottom 0.076: v41.5,16 41.75,16.25 41.75,16.7 41.45,16.99 41.45,21.79 41.99,22.33 v41.99,22.48
RESETSTATZ  (via drill 0.1 pad 0.25)
  Top 0.076: U1.C18 v42,16.5 | v46.56,22.17 46.71,22.02 51.28,22.02 53.95,19.36 v54.1,19.36 | v19.74,16.54 19.89,16.69 23.24,16.69 24.77,15.16 24.77,14.71 25.6,13.87 26.27,13.87 | U6.28 26.14,10.67 26.44,10.97 26.44,13.7 26.36,13.78 | v79.32,22.48 79.32,23.32 79.5,23.5 D6.CATHODE | 26.36,13.95 26.5,14.09 U13.B1 | 26.36,13.95 26.27,13.87 | 26.36,13.78 26.27,13.87 | 26.36,13.95 26.36,13.78
  Bottom 0.076: v19.74,16.54 19.58,16.69 19.58,18.14 22.4,20.95 37.64,20.95 38.18,21.49 38.18,24.92 38.56,25.3 42.82,25.3 43.51,24.61 46.41,24.61 46.71,24.31 46.71,22.33 v46.56,22.17 46.71,22.02 46.71,20.12 46.02,19.43 45.03,19.43 42.1,16.5 v42,16.5 | v54.1,19.36 54.1,19.89 54.63,20.42 69.57,20.42 71.78,22.63 79.17,22.63 v79.32,22.48
RGMII1_RD0
  Top 0.076: U1.U22 44,9 44,7.8 41.91,5.71 24.23,5.71 23.28,4.76 21.07,4.76 20.65,4.34 20.65,2.74 19.18,1.27 JP2.8
RGMII1_RD1
  Top 0.076: U1.V22 43.75,7.78 41.83,5.87 24.16,5.87 23.2,4.92 20.99,4.92 20.5,4.42 20.5,2.82 19.89,2.21 17.45,2.21 JP2.7
RGMII1_RD2
  Top 0.076: U1.U21 43.5,9 43.5,7.76 41.76,6.02 24.08,6.02 23.13,5.07 20.92,5.07 20.34,4.5 20.34,2.9 19.81,2.36 15.06,2.36 JP2.6
RGMII1_RD3
  Top 0.076: U1.V21 43.25,7.74 41.68,6.17 24,6.17 23.05,5.22 20.84,5.22 20.19,4.57 20.19,2.97 19.74,2.52 12.68,2.52 JP2.5
RGMII1_RX_CTL
  Top 0.076: U1.V20 42.75,7.7 41.53,6.48 23.85,6.48 22.9,5.52 20.69,5.52 19.96,4.8 18.52,4.8 18.06,4.34 18.06,3.28 17.6,2.82 7.9,2.82 JP2.3
RGMII1_RXC
  Top 0.076: U1.U20 43,9 43,7.72 41.6,6.33 23.93,6.33 22.97,5.37 20.77,5.37 20.04,4.65 20.04,3.05 19.66,2.67 10.29,2.67 JP2.4
RGMII1_TD0
  Top 0.076: U1.U25 45.5,9 45.5,7.93 42.37,4.8 27.96,4.8 27.81,4.65 27.81,2.41 JP2.11
RGMII1_TD1
  Top 0.076: U1.V25 45.25,7.91 42.29,4.95 27.89,4.95 26.75,3.81 JP3.11
RGMII1_TD2
  Top 0.076: U1.U24 45,9 45,7.89 42.22,5.11 25.68,5.11 25.22,4.65 25.22,2.36 JP2.10
RGMII1_TD3
  Top 0.076: U1.V24 44.75,7.87 42.14,5.26 25.6,5.26 24.16,3.81 JP3.10
RGMII1_TX_CTL
  Top 0.076: U1.V23 44.25,7.83 41.99,5.56 24.31,5.56 22.55,3.81 JP3.9
RGMII1_TXC
  Top 0.076: U1.U23 44.5,9 44.5,7.85 42.06,5.41 24.38,5.41 22.71,3.73 22.71,2.39 JP2.9
RGMII2_RD0  (via drill 0.1 pad 0.25)
  Top 0.076: U1.T25 v45.5,9.5
  Bottom 0.076: v45.5,9.5 45.5,7.86 43.43,5.79 43.43,5.41 43.59,5.26 44.73,5.26 45.57,4.42 45.57,2.39 JP2.18
RGMII2_RD1  (via drill 0.1 pad 0.25)
  Top 0.076: U1.R24 v45,10
  Bottom 0.076: v45,10 45.25,9.75 45.25,7.84 43.2,5.79 43.2,5.03 44.42,3.81 JP3.18
RGMII2_RD2  (via drill 0.1 pad 0.25)
  Top 0.076: U1.T24 v45,9.5
  Bottom 0.076: v45,9.5 45,7.81 43.05,5.87 43.05,2.41 JP2.17
RGMII2_RD3  (via drill 0.1 pad 0.25)
  Top 0.076: U1.R23 v44.5,10
  Bottom 0.076: v44.5,10 44.75,9.75 44.75,7.79 41.91,4.95 JP3.17
RGMII2_RX_CTL  (via drill 0.1 pad 0.25)
  Top 0.076: U1.T23 v44.5,9.5
  Bottom 0.076: v44.5,9.5 44.5,7.77 40.46,3.73 40.46,2.36 JP2.16
RGMII2_RXC  (via drill 0.1 pad 0.25)
  Top 0.076: U1.R22 v44,10
  Bottom 0.076: v44,10 44.26,9.74 44.26,7.83 41.07,4.65 40.16,4.65 39.37,3.86 JP3.16
RGMII2_TD0  (via drill 0.1 pad 0.25)
  Top 0.076: U1.T22 v44,9.5
  Bottom 0.076: v44,9.5 44,7.8 41,4.8 38.63,4.8 37.95,4.12 37.95,2.39 JP2.15
RGMII2_TD1  (via drill 0.1 pad 0.25)
  Top 0.076: U1.R21 v43.5,10
  Bottom 0.076: v43.5,10 43.75,9.75 43.75,7.78 40.92,4.95 37.95,4.95 36.83,3.83 JP3.15
RGMII2_TD2  (via drill 0.1 pad 0.25)
  Top 0.076: U1.T21 v43.5,9.5
  Bottom 0.076: v43.5,9.5 43.5,7.76 40.84,5.11 36.04,5.11 35.43,4.5 35.43,2.41 JP2.14
RGMII2_TD3  (via drill 0.1 pad 0.25)
  Top 0.076: U1.R20 v43,10
  Bottom 0.076: v43,10 43.25,9.75 43.25,7.74 40.77,5.26 35.74,5.26 JP3.14
RGMII2_TX_CTL  (via drill 0.1 pad 0.25)
  Top 0.076: U1.T20 v43,9.5
  Bottom 0.076: v43,9.5 43,7.72 40.69,5.41 33.91,5.41 32.84,4.34 32.84,2.36 JP2.13
RGMII2_TXC  (via drill 0.1 pad 0.25)
  Top 0.152: U1.R19 v42.5,10
  Bottom 0.076: v42.5,10 42.75,9.75 42.75,7.7 40.62,5.56 33.45,5.56 31.75,3.86 JP3.13
RXD  (via drill 0.1 pad 0.25)
  Top 0.076: JP1.2 30.15,25.07 32.23,25.07 33.05,24.25 U12.B1 v33.78,24 | v37.47,21.84 R76.2
  Bottom 0.076: v33.78,24 34.21,23.57 34.21,23.01 35.2,22.02 36.5,22.02 36.77,22.29 37.19,22.29 37.47,22.01 v37.47,21.84
SD_LS_ON
  Top 0.127: D7.ANODE D6.ANODE | R54.2 81.18,22.45 D6.ANODE | U10.3 82.11,24.03 81.57,23.5 D6.ANODE
SDCD_INV  (via drill 0.1 pad 0.25, 0.25 pad 0.46)
  Top 0.076: U11.2 88.9,5.46 88.77,5.33 87.76,5.33 87.63,5.46 R48.1 87.17,5.92 v86.74,6.35
  Top 0.127: X1.PIN10 86.23,15.94 v86.23,11.68 86.23,10.32 X1.PIN9
  Bottom 0.127: v86.74,6.35 86.74,11.18 v86.23,11.68
SPI0_CLK  (via drill 0.1 pad 0.25)
  Top 0.076: U1.C11 v38,16.5 | v37.19,19.05 37.34,19.2 38.41,19.2 39.32,20.12 40.62,20.12 41.07,20.57 41.07,21.18 43.74,23.85 52.05,23.85 54.56,21.34 57.07,21.34 57.38,21.64 58.22,21.64 v58.67,21.18
  Bottom 0.076: v38,16.5 38,18.08 37.19,18.9 v37.19,19.05 | v58.67,21.18 58.83,21.03 69.27,21.03 71.48,23.24 84.2,23.24 86.49,25.53 91.59,25.53 92.71,26.64 JP4.37
SPI0_CS0  (via drill 0.1 pad 0.25)
  Top 0.076: U1.D13 v39,16 | v58.29,21.18 57.99,20.88 54.33,20.88 51.82,23.39 43.97,23.39 41.53,20.95 41.53,20.34 40.84,19.66 39.55,19.66 38.63,18.75 38.48,18.75 v38.33,18.59
  Bottom 0.076: v39,16 38.75,16.25 38.75,18.02 38.33,18.44 v38.33,18.59 | v58.29,21.18 58.6,20.88 69.34,20.88 71.55,23.09 84.28,23.09 86.56,25.38 93.95,25.38 JP4.38
SPI0_CS1  (via drill 0.1 pad 0.25)
  Top 0.076: U1.C13 v39,16.5
  Bottom 0.076: v39,16.5 U1.C13 39.25,15.88 39.12,15.75 36.88,15.75 36.75,15.62 36.75,14.75 36.48,14.48 33.98,14.48 32.69,15.77 32.69,17.07 32,17.75 23.01,17.75 21.41,16.15 21.41,14.55 20.12,13.26 15.85,13.26 15.01,12.42 15.01,6.02 14.4,5.41 10.9,5.41 10.59,5.11 5.11,5.11 JP3.2
SPI0_D0  (via drill 0.1 pad 0.25)
  Top 0.076: U1.D12 v38.5,16 | v37.57,18.9 37.72,19.05 38.48,19.05 39.4,19.96 40.69,19.96 41.22,20.5 41.22,21.11 43.81,23.7 51.97,23.7 54.48,21.18 57.15,21.18 57.45,21.49 57.61,21.49 v57.91,21.18
  Bottom 0.076: v38.5,16 38.25,16.25 38.25,18.06 37.57,18.75 v37.57,18.9 | v57.91,21.18 58.6,21.87 61.57,21.87 62.18,22.48 70.48,22.48 71.4,23.39 84.12,23.39 86.41,25.68 89.23,25.68 90.17,26.62 JP4.36
SPI0_D1  (via drill 0.1 pad 0.25)
  Top 0.076: U1.C12 v38.5,16.5 | v57.53,21.18 57.38,21.03 54.41,21.03 51.89,23.55 43.89,23.55 41.38,21.03 41.38,20.42 40.77,19.81 39.47,19.81 38.56,18.9 38.1,18.9 v37.95,18.75
  Bottom 0.076: v38.5,16.5 38.5,18.04 37.95,18.59 v37.95,18.75 | v57.53,21.18 58.37,22.02 61.49,22.02 62.1,22.63 70.41,22.63 71.32,23.55 84.05,23.55 87.17,26.67 JP4.35
TCK  (via drill 0.1 pad 0.25, 0.25 pad 0.46)
  Top 0.076: U1.D9 v37,16 | v20.65,17.98 20.5,17.83 19.81,17.83 19.2,18.44 17.88,18.44 17.5,18.06 17.12,18.06 R19.1
  Top 0.127: R19.1 17.02,18.11 v17.02,18.8 16.38,19.43 TC1.4
  Bottom 0.076: v37,16 36.75,16.25 36.75,18.19 36.04,18.9 23.16,18.9 22.55,19.51 22.1,19.51 21.26,18.67 21.26,18.14 21.11,17.98 v20.65,17.98
TDI  (via drill 0.1 pad 0.25, 0.25 pad 0.46)
  Top 0.076: U1.D10 v37.5,16 | v23.24,19.58 23.47,19.81 23.47,20.88 21.26,23.09 18.44,23.09 17.22,24.31 14.86,24.31 14.55,24 14.55,23.65 R17.1
  Top 0.127: TC1.8 15.11,22.35 v14.61,22.86 14.61,23.55 R17.1
  Bottom 0.076: v37.5,16 37.25,16.25 37.25,18.15 36.2,19.2 23.62,19.2 v23.24,19.58
TDO  (via drill 0.1 pad 0.25, 0.25 pad 0.46)
  Top 0.076: U1.D11 v38,16 | v22.86,20.19 22.86,21.03 21.11,22.78 17.73,22.78 v17.65,22.86
  Top 0.127: TC1.6 v17.65,22.86
  Bottom 0.076: v38,16 37.75,16.25 37.75,18.11 36.35,19.51 24,19.51 23.32,20.19 v22.86,20.19
TMS  (via drill 0.1 pad 0.25, 0.25 pad 0.46)
  Top 0.076: U1.C10 v37.5,16.5 | R18.1 14.86,17.98 15.24,17.98 15.58,17.64 20.65,17.64 20.95,17.95 v20.95,18.29
  Top 0.127: TC1.2 v13.84,18.8 14.1,18.54 14.61,18.54 14.73,18.41 14.73,18.11 R18.1
  Bottom 0.076: v37.5,16.5 37.5,18.13 36.27,19.36 23.93,19.36 23.39,19.89 22.25,19.89 20.95,18.59 v20.95,18.29
TPS22965_CT
  Top 0.127: U5.6 13.59,6.48 13.72,6.6 C28.1
TPS22965_EN  (via drill 0.1 pad 0.25)
  Top 0.127: U6.17 15.78,8.45 15.71,8.38 v14.4,8.38 | R73.1 9.14,5.41 v9.53,5.41 | U5.3 v9.53,6.48
  Bottom 0.127: v9.53,6.48 v9.53,5.41 10.59,5.41 10.82,5.64 14.17,5.64 14.4,5.87 v14.4,8.38
TRSTN  (via drill 0.1 pad 0.25, 0.25 pad 0.46)
  Top 0.076: U1.C9 v37,16.5 | v23.24,19.2 23.62,19.58 23.62,20.95 21.34,23.24 18.52,23.24 17.3,24.46 12.57,24.46 12.27,24.16 12.27,23.65 R14.2
  Top 0.127: R14.2 12.32,23.55 v12.32,22.86 12.83,22.35 13.59,22.35 13.84,22.1 TC1.9
  Bottom 0.076: v37,16.5 37,18.17 36.12,19.05 23.39,19.05 v23.24,19.2
TS_INT#  (via drill 0.1 pad 0.25)
  Top 0.076: U13.D2 27.2,12.99 27.2,11.58 v27.36,11.43
  Bottom 0.076: J8.9 23.46,7.38 23.77,7.7 24,7.7 27.2,10.9 27.2,11.28 v27.36,11.43 27.36,11.61 TP7.TP
TS_RESET_N  (via drill 0.1 pad 0.25)
  Top 0.076: v26.9,11.43 27.05,11.58 27.05,13.34 U13.C2
  Bottom 0.076: J8.8 22.96,7.49 23.32,7.85 23.93,7.85 27.05,10.97 27.05,11.28 v26.9,11.43 26.9,11.58 TP6.TP
TXD
  Top 0.076: U12.C1 33.17,23.75 32.79,24.13 JP1.3
UART0_CTSN  (via drill 0.1 pad 0.25)
  Top 0.076: U1.A9 37.25,17.84 36.5,18.59 36.5,22.1 36.69,22.29 36.92,22.29 37.07,22.44 37.07,22.82 v37.19,22.94
  Bottom 0.076: v37.19,22.94 37.03,23.09 37.03,25.22 38.48,26.67 JP4.16
UART0_RTSN  (via drill 0.1 pad 0.25)
  Top 0.076: U1.B9 37,17 37,17.86 36.35,18.52 36.35,22.25 36.65,22.55 v36.8,22.55
  Bottom 0.076: v36.8,22.55 36.88,22.63 36.88,25.3 38.18,26.59 38.18,28.04 39.34,29.21 JP5.16
UART0_RXD  (via drill 0.1 pad 0.25)
  Top 0.076: U1.A10 37.75,17.8 36.8,18.75 36.8,21.34 37.11,21.64 37.11,21.87 v36.96,22.02 | U12.C2 v33.78,23.5
  Bottom 0.076: v36.96,22.02 36.73,22.02 36.58,21.87 35.13,21.87 34.06,22.94 34.06,23.22 v33.78,23.5
UART0_TXD  (via drill 0.1 pad 0.25)
  Top 0.076: U1.B10 37.5,17 37.5,17.82 36.65,18.67 36.65,21.57 v36.8,21.72 | U12.D2 34.03,23.24 v33.78,22.99
  Bottom 0.076: v36.8,21.72 35.05,21.72 v33.78,22.99
USB0_CC1
  Top 0.127: J5.A5 7.38,16.51 R35.2
USB0_CC2
  Top 0.127: R36.2 9.19,13.49 J5.B5
USB0_DM  (via drill 0.1 pad 0.25, 0.25 pad 0.46)
  Top 0.076: U1.U12 39,9 39,8.55 39.24,8.31 39.24,7.16 38.71,6.63 29.18,6.63 28.65,7.16 28.65,13.79 26.75,15.7 24.54,15.7 23.32,16.92 19.74,16.92 19.58,16.76 19.28,16.76 v19.13,16.61
  Top 0.127: v6.35,14.86 6.48,14.99 J5.A7 8.13,14.99 8.26,15.11 8.38,15.11 v8.64,14.86 8.89,15.11 9.15,15.11 9.28,14.99 U9.2 | J5.B7 6.62,15.99 v6.35,16.26
  Bottom 0.076: v8.64,14.86 8.94,15.16 10.9,15.16 13.11,17.37 18.36,17.37 18.52,17.22 18.52,16.92 18.67,16.76 18.97,16.76 v19.13,16.61
  Bottom 0.127: v6.35,14.86 5.84,15.37 5.84,15.75 v6.35,16.26
USB0_DP  (via drill 0.1 pad 0.25, 0.25 pad 0.46)
  Top 0.076: U1.V12 38.75,8.57 39.09,8.23 39.09,7.24 38.63,6.78 29.26,6.78 28.8,7.24 28.8,13.87 26.82,15.85 24.61,15.85 23.39,17.07 19.66,17.07 19.51,16.92 19.28,16.92 v19.13,17.07
  Top 0.127: J5.B6 6.62,14.49 v6.35,14.22 | v6.35,15.62 6.48,15.49 J5.A6 8.13,15.49 8.26,15.37 8.38,15.37 v8.64,15.62 8.89,15.37 9.14,15.37 9.26,15.49 U9.1
  Bottom 0.076: v8.64,15.62 8.94,15.32 9.3,15.32 9.37,15.39 9.37,15.7 9.45,15.77 9.68,15.77 9.75,15.7 9.75,15.39 9.83,15.32 10.82,15.32 13.03,17.53 18.44,17.53 18.67,17.3 18.67,16.99 18.75,16.92 18.97,16.92 v19.13,17.07
  Bottom 0.127: v6.35,14.22 6.86,14.73 6.86,15.11 v6.35,15.62
USB0_DRVVBUS  (via drill 0.1 pad 0.25)
  Top 0.076: U1.C19 v42.5,16.5 | J4.11 69.04,11.05 68.43,11.66 57,11.66 49.84,18.82 46.63,18.82 46.18,19.28 45.49,19.28 v45.34,19.13
  Bottom 0.076: v42.5,16.5 42.5,16.67 44.96,19.13 v45.34,19.13
USB0_VBUS
  Top 0.076: U1.V11 38.25,8.61 38.79,8.08 38.79,7.39 38.48,7.09 29.57,7.09 29.18,7.47 29.18,14.02 26.98,16.23 24.77,16.23 23.51,17.49 14.59,17.49 14.12,17.02 R62.1
  Top 0.127: R63.1 13.59,17.98 13.59,17.07 R62.1
USB1_CC1  (via drill 0.1 pad 0.25)
  Top 0.076: J6.A5 65.3,20.41 v65.3,19.74 | R72.1 59.56,19.56 59.28,19.28 v58.9,19.28
  Bottom 0.076: v65.3,19.74 65.08,19.96 63.93,19.96 63.7,19.74 63.7,19.2 63.55,19.05 59.13,19.05 v58.9,19.28
USB1_CC2  (via drill 0.1 pad 0.25)
  Top 0.076: J6.B5 66.8,18.68 v66.8,18.03 | v58.52,19.28 58.52,20.42 59.16,21.06 R71.1
  Bottom 0.076: v66.8,18.03 65.94,18.9 58.9,18.9 v58.52,19.28
USB1_DM  (via drill 0.1 pad 0.25)
  Top 0.076: J6.A7 66.29,19.96 66.14,19.81 66.14,19.66 66.29,19.51 67.51,19.51 68.05,18.97 68.05,18.75 v68.2,18.59 68.05,18.44 68.05,18.14 67.51,17.6 66.22,17.6 65.99,17.83 65.99,18.06 65.84,18.21 65.84,18.65 J6.B7 | v58.14,18.44 58.29,18.59 58.52,18.59 58.67,18.44 58.89,18.44 U2.2 | U1.U10 38,9 38,8.56 38.1,8.46 38.1,7.92 38.18,7.85 38.33,7.85 v38.48,8
  Route15 0.076: v52.43,12.62 52.27,12.47 52.05,12.47 51.89,12.32 51.89,11.81 48.77,8.69 39.4,8.69 39.09,8.38 39.09,8.08 38.86,7.85 38.63,7.85 v38.48,8
  Bottom 0.076: v52.43,12.62 52.27,12.47 52.05,12.47 51.89,12.62 51.89,14.02 53.87,16 53.87,16.84 55.63,18.59 57.99,18.59 v58.14,18.44 58.29,18.59 65.38,18.59 66.37,17.6 67.51,17.6 68.05,18.14 68.05,18.44 v68.2,18.59
USB1_DP  (via drill 0.1 pad 0.25)
  Top 0.076: J6.A6 65.84,20.38 65.84,19.96 65.99,19.81 65.99,19.58 66.22,19.36 67.44,19.36 67.89,18.9 67.89,18.75 v67.74,18.59 67.89,18.44 67.89,18.21 67.44,17.75 66.29,17.75 66.14,17.91 66.14,18.06 66.29,18.21 J6.B6 | v58.14,18.9 58.29,18.75 58.52,18.75 58.64,18.86 U2.1 | v38.48,7.54 38.33,7.7 38.1,7.7 37.95,7.85 37.95,8.38 37.75,8.58 U1.V10
  Route15 0.076: v52.43,12.17 52.27,12.32 52.12,12.32 52.05,12.24 52.05,11.73 48.84,8.53 39.48,8.53 39.24,8.29 39.24,8 38.94,7.7 38.63,7.7 v38.48,7.54
  Bottom 0.076: v52.43,12.17 52.27,12.32 51.97,12.32 51.74,12.55 51.74,14.1 53.72,16.08 53.72,16.92 55.55,18.75 57.99,18.75 v58.14,18.9 58.29,18.75 65.46,18.75 66.45,17.75 67.44,17.75 67.89,18.21 67.89,18.44 v67.74,18.59
USB1_DRVVBUS  (via drill 0.1 pad 0.25)
  Top 0.076: U1.D19 v42.5,16 | J4.12 70.04,11.27 69.49,11.81 57.07,11.81 49.91,18.97 46.71,18.97 46.18,19.51 45.34,19.51 45.03,19.2 45.03,18.97 45.19,18.82 45.57,18.82 v45.72,18.97
  Bottom 0.076: v42.5,16 42.75,16.25 42.75,16.69 44.88,18.82 45.57,18.82 v45.72,18.97
USB1_VBUS
  Top 0.076: U1.U11 38.5,9 38.5,8.59 38.94,8.15 38.94,7.32 38.56,6.93 29.49,6.93 29.03,7.39 29.03,13.95 26.9,16.08 24.69,16.08 23.43,17.34 14.67,17.34 14.4,17.07 14.4,16.31 14.1,16 R5.1
  Top 0.127: R4.1 13.59,15.04 13.59,15.95 R5.1
VBUS  (via drill 0.1 pad 0.25)
  Top 0.254: C60.1 9.02,21.59 v8.89,21.72 | D8.A v6.73,21.59 | C50.1 11.37,15.49 U9.6 10.28,15.51 9.78,16 9.78,17.02 9.16,17.64 J5.A4_B9
  other vias: 5.84,13.08 6.22,13.08 6.22,13.46 5.84,13.46 5.84,13.84 5.84,17.4 6.22,17.4 6.22,17.02 5.84,17.02 5.84,16.64 8.51,22.1 8.89,22.1 8.51,21.72 6.73,21.21 6.73,21.97
  pour Bottom: 3.81,12.95 6.35,12.95 6.35,13.46 5.46,14.35 5.46,16.13 6.35,17.02 6.35,17.53 5.33,17.53 5.33,20.19 5.97,20.83 9.27,20.83 9.27,22.35 3.81,22.35
  pour Top (no thermals): 8,17.91 8,17.4 6.73,17.4 5.71,16.38 5.71,17.53 6.55,17.53 6.93,17.91
  pour Top (no thermals): 8,12.57 8,13.08 6.73,13.08 5.71,14.1 5.71,12.95 6.55,12.95 6.93,12.57
  pour Top (no thermals): 6.48,22.35 6.48,20.83 9.27,20.83 9.27,22.35
VDD1P8_CAP
  Top 0.254: U6.14 14.49,10.17 14.22,9.91 C41.1
VDD_SD
  Top 0.508: X1.PIN4 96.66,13.84 89.53,13.84 88.77,14.61 88.77,20.42 87.76,21.43 U10.6
  pour Top (no thermals): 86.87,20.45 86.87,25.15 85.47,25.15 85.47,21.97 83.06,21.97 83.06,20.45
VIN-3P3  (via drill 0.1 pad 0.25, 0.25 pad 0.46)
  Top 0.127: R9.1 C30.2 R73.2 9.02,6.3 9.3,6.02 10.15,6.02 U5.4 | C48.1 21.51,8.64 R22.2
  Top 0.254: U6.13 v14.35,10.67 | U6.4 v17.78,14.22 18.16,14.61 C52.1 | U6.5 17.28,14.09 v17.14,14.22 C51.1 | U6.6 16.78,13.83 v16.38,14.22 16.13,14.48 C40.1 | U6.22 18.28,7.92 v18.49,7.67 18.8,7.37 C39.1 | U6.26 20.53,9.67 v20.57,9.63 20.57,8.89 20.83,8.64 C48.1 | U6.30 20.49,11.67 v20.57,11.76
  Bottom 0.381: v18.49,7.67 18.72,7.67 20.57,9.53 v20.57,9.63
  other vias: 10.9,10.06 10.9,10.44 11.28,10.44 11.28,10.06 10.9,9.68 11.28,9.68
  pour Top (no thermals): 10.46,6.96 9.14,6.96 9.14,6.48 8.51,6.48 8.51,8.13 9.4,8.13 9.4,10.41 10.03,10.41 10.03,12.95 11.43,12.95 11.43,9.65 10.46,9.65
  pour Route15 (isolate 0.127): 20.95,14.61 16.64,14.61 14.86,12.83 14.1,12.83 12.19,10.92 10.03,10.92 10.03,9.53 20.95,9.53
VIN-3P3-LS  (via drill 0.1 pad 0.25, 0.25 pad 0.46)
  Top 0.076: U1.B15 v40.5,17 | R32.2 v71.5,6.22 | R31.2 v72.52,6.22 | R30.2 v73.53,6.22 | R28.2 v75.56,6.22 | R7.2 v94.61,24.13 | U11.6 88.55,7.39 v88.39,7.54 87.76,7.54 87.63,7.42 R48.2 | R10.2 33.4,21.31 v33.15,21.57 | U12.A2 v33.78,24.51 U12.B2 | C61.1 34.04,22.56 v34.04,22.1 | U13.B2 U13.A2 27.3,14.76 v26.9,15.16 | R11.2 v42.67,24.13
  Top 0.127: R13.2 12.45,11 12.45,11.86 R25.2 12.45,12.01 12.45,12.88 R52.2 12.45,13.03 12.45,13.89 R53.2 | TC1.1 v12.57,18.8 | R21.2 8.76,23.55 v8.76,22.99 | R17.2 13.34,23.55 v13.34,22.86 | R20.2 15.62,23.55 v15.62,22.86 | R18.2 16,18.11 v16,18.8 | R19.2 v18.92,18.03 | R38.2 v77.72,21.34 | R49.2 v72.64,21.34 | R51.2 v71.63,21.34 | J4.15 73.03,9.42 | C29.1 12.37,9.02 v12.95,9.02 | U5.7 12.19,7.01 12.19,7.45 U5.8 12.19,7.51 v12.19,8.13 | v71.25,17.65 U4.4 | U8.1 76.41,17.78 v75.82,17.78 | v75.82,17.14 75.39,17.14 C26.1 | v74.55,20.7 75.13,20.7 C35.1 | v79.88,20.7 79.88,21.26 R16.2 79.88,21.41 79.88,22.28 R54.1 | C36.1 v79.63,10.41 79.63,9.73 R12.2 79.63,9.58 79.63,8.71 R64.2 | v21.95,13.56 21.67,13.56 R23.2 | v1.14,9.65 1.14,9.01 U7.1 | C34.1 9.4,18.03 v9.22,18.21 | C22.1 50.04,13.28 50.04,13.72 50.29,13.97 C6.1 | R57.2 v3.3,22.73
  Top 0.152: U1.N11 v38,11 | U1.P10 v37.5,10.5 | U1.M21 v43.5,11.5 | U1.M22 v44,11.5 | U1.L21 v43.5,12 | U1.L22 v44,12 | U1.G10 v37.5,14.5 | U1.G11 v38,14.5 | U1.F11 v38,15 | U1.F12 v38.5,15 | U1.J22 v44,13.5 | U1.J21 v43.5,13.5 | U1.H21 v43.5,14 | U1.H22 v44,14 | U1.N7 v36,11 | U1.K21 v43.5,12.5 | U1.K22 v44,12.5 | R66.2 v35.43,25.27 | R65.2 v36.45,25.27
  Top 0.254: R53.2 12.06,13.97 v11.81,13.72 | 73.03,9.42 v73.03,10.79 78.19,10.79 C37.1 | R13.2 12.06,10.92 11.94,11.05 v11.94,11.43 | v50.04,12.57 50.04,13.13 C22.1 | C63.1 v40.26,20.95 40.39,20.95 41.3,21.87 41.3,22.64 U14.4 41.53,22.86 v41.99,22.86
  Top 0.508: JP4.34 84.39,25.97 U10.1
  Route15 0.254: v37.5,10.5 v38,11
  Bottom 0.127: R68.2 v13.97,22.86 | R67.2 11.43,23.11 v11.68,22.86 | v87.63,9.65 R70.2 | R69.2 v90.17,9.65
  Bottom 0.152: v37.5,10.5 36.5,10.5 v36,11 | v41.5,11 40.5,11 v40,11.5
  Bottom 0.254: v44,12 v44,12.5 43.94,12.5 | v44,12 v44,11.5 v43.5,11.5 | v44,13.5 v44,14 v43.5,14 | v44,13.5 v43.5,13.5 | 43.94,12.5 v43.5,12.5 | v44,12 v43.5,12 | v44,13.5 44,12.56 43.94,12.5 | J8.1 19.46,5.87 19.18,5.59 v19.18,5.31
  other vias: 12.95,7.11 12.95,7.75 12.95,8.38
  pour Top (no thermals): 11.94,6.86 11.94,9.14 13.21,9.14 13.21,6.86
  pour Route15 (isolate 0.127, rank 6): -7.62,38.1 109.22,38.1 109.22,-7.62 -7.62,-7.62
VIN-5P0  (via drill 0.1 pad 0.25, 0.25 pad 0.46)
  Top 0.127: 64.77,18.71 J6.B9 64.77,18.67 | 64.77,20.4 J6.A4 64.77,20.44 | v4.32,24.13 4.38,24.19 9.21,24.19 9.4,24 9.4,22.73 9.65,22.48 9.65,19.43 10.54,18.54 10.54,17.4 10.92,17.02 R62.2 12.45,16.94 12.45,16.08 R5.2 | R2.2 48.01,24.64 48.13,24.77 48.13,27.94
  Top 0.254: J6.B4 v67.28,18.01 | J6.A9 v67.28,19.76 | C24.1 60.73,19.96 R72.2 | R71.2 60.73,21.01 | 60.73,21.01 C24.1 | C24.1 60.67,18.86 U2.6 | v64.14,19.56 64.75,19.56 64.77,19.58 | 63.5,23.5 63.34,23.5 62.74,22.89 61.63,22.89 60.73,22 60.73,21.01 | C59.1 v4.88,24.64 C55.1 | C56.1 v4.32,23.37 | D8.C 4.32,21.87 v4.32,22.99
  Top 0.508: v33.02,27.56 33.4,27.94 48.13,27.94 62.87,27.94 63.5,27.3 63.5,23.5 64.77,22.23 64.77,20.44 | 64.77,20.4 64.77,19.58 64.77,18.71 | 64.77,18.67 v64.77,17.14 v65.53,17.14 | JP3.34 85.09,6.1 v85.85,6.86
  Bottom 0.254: v67.28,19.76 67.28,19.28 | 67.28,19.28 v67.28,18.01 | v64.14,19.56 64.41,19.28 67.28,19.28
  Bottom 0.508: v85.85,6.86 83.57,6.86 81.15,9.27 66.04,9.27 64.77,10.54 v64.77,17.14 | v33.4,28.19 33.15,27.94 16.51,27.94 | 16.51,27.94 5.59,27.94 5.08,27.43 5.08,24.84 v4.88,24.64 | JP4.7 16.51,27.94 | JP2.1 2.54,2.54 2.54,5.82 4.95,8.23 v4.95,10.92
  other vias: 3.94,23.37 3.94,22.99 85.85,7.49 65.15,17.65 32.64,28.19 85.85,6.22 4.32,23.75 4.7,11.18 5.21,11.18 5.21,10.67 4.7,10.67 3.94,23.75 3.94,24.13
  pour Top (no thermals): 3.81,9.78 4.57,9.02 5.31,9.02 5.31,9.65 7.49,9.65 7.49,10.03 5.33,10.03 5.33,20.19 5.97,20.83 5.97,25.27 3.81,25.27
  pour Bottom: 3.81,25.27 5.97,25.27 5.97,22.86 3.81,22.86
  pour Bottom: 32.38,28.19 32.77,28.57 33.27,28.57 33.66,28.19 33.66,27.69 33.27,27.3 32.77,27.3 32.38,27.69
  pour Top: 32.77,28.57 33.27,28.57 33.66,28.19 33.66,27.69 33.27,27.3 32.77,27.3 32.38,27.69 32.38,28.19
  pour Top (no thermals): 83.31,5.21 86.23,5.21 86.23,7.8 83.31,7.8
